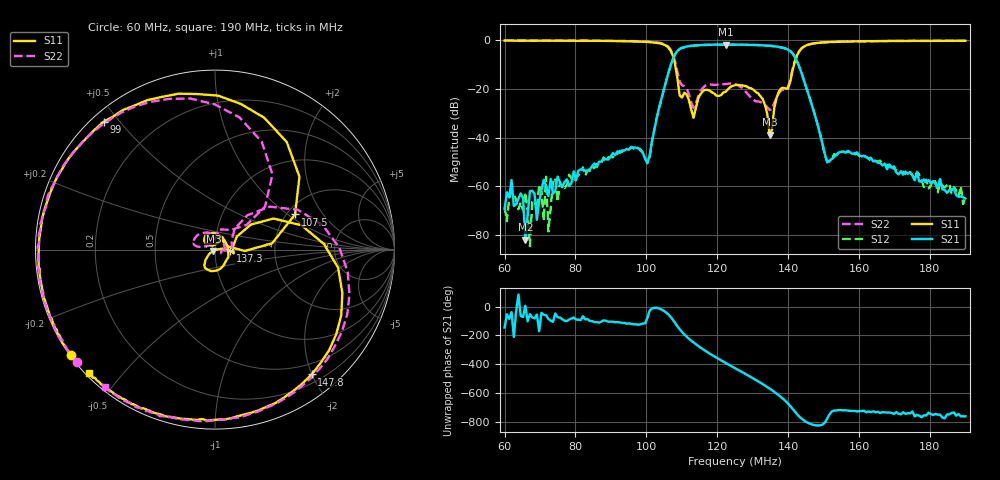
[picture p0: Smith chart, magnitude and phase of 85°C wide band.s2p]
!Agilent Technologies,E8362C,SG49020144,A.09.33.09
!Agilent E8362C: A.09.33.09
!Date: Friday, October 10, 2025 09:08:38
!Correction: S11(Full 2 Port(1,2))
!S21(Full 2 Port(1,2))
!S12(Full 2 Port(1,2))
!S22(Full 2 Port(1,2))
!S2P File: Measurements: S11, S21, S12, S22:
# Hz S  dB  R 50
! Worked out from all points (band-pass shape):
!   201 points, 60 MHz to 190 MHz, reference 50 ohm
!   highest |S21| = -1.69 dB at 122.4 MHz (marker M1); lowest = -82.0 dB at 65.85 MHz (marker M2)
!   |S21| within 3 dB of the highest: 108.6 MHz to 140.8 MHz (32.23 MHz wide, 25.9 % of centre)
!   lowest |S11| = -38.8 dB at 134.8 MHz (marker M3), VSWR 1.02, Z = 49.1 - j0.719 ohm
!   |S11| at or under -10 dB: 108.1 MHz to 141.7 MHz (33.55 MHz wide, 26.9 % of centre)
!   |S22| runs from -28.6 to 0.0 dB; largest |S21 - S12| = 0.008
!   S11 on the Smith chart (normalised r, x): 60 MHz: 0.00, -0.33; 99 MHz: 0.03, +0.46; 107.5 MHz: 2.21, +1.13; 137.3 MHz: 1.19, -0.02; 147.8 MHz: 0.32, -2.00; 190 MHz: 0.01, -0.41
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6e7  -0.05 -143.8  -69.44 -144.5  -68.68 -36.4  -0.06 -140.9
6.195e7  -0.05 -146.5  -57.45 -38.1  -62.14 -33.0  -0.05 -143.7
6.585e7  -0.06 -152.0  -82.02 6.1  -62.52 -46.6  -0.08 -148.7
6.715e7  -0.06 -154.1  -62.02 -52.7  -84.70 108.3  -0.03 -150.5
7.105e7  -0.09 -159.8  -57.34 -56.3  -74.15 -90.1  -0.03 -155.9
7.17e7  -0.11 -161.0  -59.85 -59.3  -56.08 -48.3  -0.05 -156.9
7.235e7  -0.10 -162.1  -64.03 -84.2  -78.66 -61.2  -0.05 -157.8
7.365e7  -0.09 -163.9  -63.14 -105.8  -57.42 -51.7  -0.08 -159.8
8.21e7  -0.15 -178.3  -53.19 -66.6  -52.23 -104.8  -0.08 -172.9
9.9e7  -0.49 131.0  -46.35 -117.3  -46.16 -119.3  -0.42 143.1
1.0355e8  -1.18 96.6  -27.95 -12.5  -28.08 -13.5  -0.93 113.7
1.0745e8  -6.25 23.7  -7.74 -90.2  -7.80 -90.4  -5.57 52.6
1.146e8  -24.04 145.7  -2.00 87.7  -1.98 87.6  -23.15 168.7
1.224e8  -21.12 -46.4  -1.69 -30.9  -1.71 -31.0  -17.93 159.4
1.25e8  -18.46 -93.4  -1.74 -66.5  -1.73 -66.5  -17.94 140.3
1.3475e8  -38.83 -140.2  -2.22 152.1  -2.19 152.3  -28.63 -22.9
1.3735e8  -21.25 -4.3  -2.69 105.6  -2.69 105.4  -21.72 9.0
1.471e8  -1.27 -47.4  -28.56 -99.8  -28.53 -99.6  -1.34 -38.8
1.4775e8  -1.11 -52.2  -31.85 -102.6  -31.82 -102.2  -1.17 -44.1
1.51e8  -0.71 -71.8  -50.20 -56.4  -49.54 -59.6  -0.77 -64.0
1.6855e8  -0.22 -115.0  -51.04 -13.6  -51.38 -25.2  -0.19 -108.4
1.9e8  -0.16 -135.6  -65.08 -40.5  -64.70 -60.0  -0.15 -128.6
